(* Logix 5000 AddOnInstructionDefinition export Banner_IOL_QM30VT3_Parameter_v5; software revision 33.00 *)

TYPE Banner_IOL_Device_SubIndex :
STRUCT
   Sub : DINT[34];
END_STRUCT
END_TYPE

TYPE Banner_IOL_Port_v5 :   // UDT that has all of the data items necessary to communicate with a specific Port on a IO-Link Master
STRUCT
   Port_Controlled : INT;   // Each bit represents a port on an IO-Link Master. Set to 1 to tell AOI to control that port.
   Port_Activate : INT;   // Each bit represents a port on an IO-Link Master. When ON that port will process any commands in queue.
   Port_Read : INT;   // Each bit represents a port on an IO-Link Master. Used to determine when device AOI has requested a Read command.
   Port_Write : INT;   // Each bit represents a port on an IO-Link Master. Used to determine when device AOI has requested a Write command.
   Port_RW_Complete : INT;   // Each bit represents a port on an IO-Link Master. Tells device AOI that Read or Write request has been completed.
   Port_Device_Read : INT;
   Data_Transfer : SINT[250];   // Array to transfer data from IO-Master to device AOIs.
END_STRUCT
END_TYPE

TYPE Banner_IOL_QM30VT3_Device :
STRUCT
   Initial_Global_Read : BOOL;
   Command : SINT;
   Data : Banner_IOL_QM30VT3_Device_Index;
   Reset : BOOL;
END_STRUCT
END_TYPE

TYPE Banner_IOL_QM30VT3_Device_Index :
STRUCT
   Index : Banner_IOL_Device_SubIndex[19];
   Metric_Config : Banner_IOL_QM30VT3_Metric_Config;
END_STRUCT
END_TYPE

TYPE Banner_IOL_QM30VT3_Metric_Config :
STRUCT
   Metric_1 : Banner_IOL_QM30VT3_Metric_Data;
   Metric_2 : Banner_IOL_QM30VT3_Metric_Data;
   Metric_3 : Banner_IOL_QM30VT3_Metric_Data;
   Metric_4 : Banner_IOL_QM30VT3_Metric_Data;
   Metric_5 : Banner_IOL_QM30VT3_Metric_Data;
   Metric_6 : Banner_IOL_QM30VT3_Metric_Data;
   Metric_7 : Banner_IOL_QM30VT3_Metric_Data;
   Num_of_Threshold_Samples : DINT;
END_STRUCT
END_TYPE

TYPE Banner_IOL_QM30VT3_Metric_Data :
STRUCT
   Metric : DINT;   // See IODD file for all options.
   Warning_Threshold : REAL;
   Alarm_Treshold : REAL;
END_STRUCT
END_TYPE

TYPE Banner_IOL_Rules :
STRUCT
   Byte_Pos : SINT;   // Byte Position to read from or write data to.
   Multi : SINT;   // Determines if a multiple byte length index is being accessed. Use 2 for 2 bytes length, 3 for 3 byte length, etc..
   Sub_Index : SINT;
   Signed : SINT;   // 0=Unsigned, 1=Signed
END_STRUCT
END_TYPE

TYPE Banner_IOL_Rules_Array :
STRUCT
   Length : DINT;
   Settings : Banner_IOL_Rules_SettingsArray[32];
END_STRUCT
END_TYPE

TYPE Banner_IOL_Rules_SettingsArray :
STRUCT
   Index : DINT;
   Num_Op : INT;   // Number of Operations to read/write Index.
   Total_Bytes : INT;
   RW : SINT;   // 0 = Read Only, 1 = Write Only, 2 = Read or Write
   Rules : Banner_IOL_Rules[34];   // Sub Index Position in IODD.
END_STRUCT
END_TYPE

ADD_ON_INSTRUCTION Banner_IOL_QM30VT3_Parameter_v5   (* revision 5.0 *)
// AOI that reads and writes to an IO-Link devices parameter data.
VAR_IN_OUT
   Device : Banner_IOL_QM30VT3_Device; {required}
   Rules : Banner_IOL_Rules_Array; {required}
   Port_Data : Banner_IOL_Port_v5; {required}
END_VAR
VAR_INPUT
   Port : DINT; {required}
END_VAR
VAR_OUTPUT
   Done : BOOL; {access Read Only, visible}
   Busy : BOOL; {access Read Only, visible}
END_VAR
VAR
   Control : DINT; {access None}
   Inprocess_Index : INT; {access None}
   Index_Write_Inprocess : INT; {access None}
   Index_Write_Control : INT; {access None}
   Global_Read_Command : INT; {access None}
   Command_Being_Processed : BOOL; {access None}
   r_dex2 : INT; {access None}
   r_dex1 : INT; {access None}
   g_index : INT; {access None}
   r_dex3 : INT; {access None}
   r_dex4 : INT; {access None}
   r_dex5 : INT; {access None}
   Wr_Upper : INT; {access None}
   w_dex5 : INT; {access None}
   w_dex4 : INT; {access None}
   w_dex3 : INT; {access None}
   w_dex2 : INT; {access None}
   w_dex1 : INT; {access None}
   m3 : INT; {access None}
   m2 : INT; {access None}
   m1 : INT; {access None}
   s_dex : INT; {access None}
   GlobalCon : DINT; {access None}
   b_dex : INT; {access None}
   Temp_Int : INT; {access None}
END_VAR

ROUTINE Logic   (* ladder *)
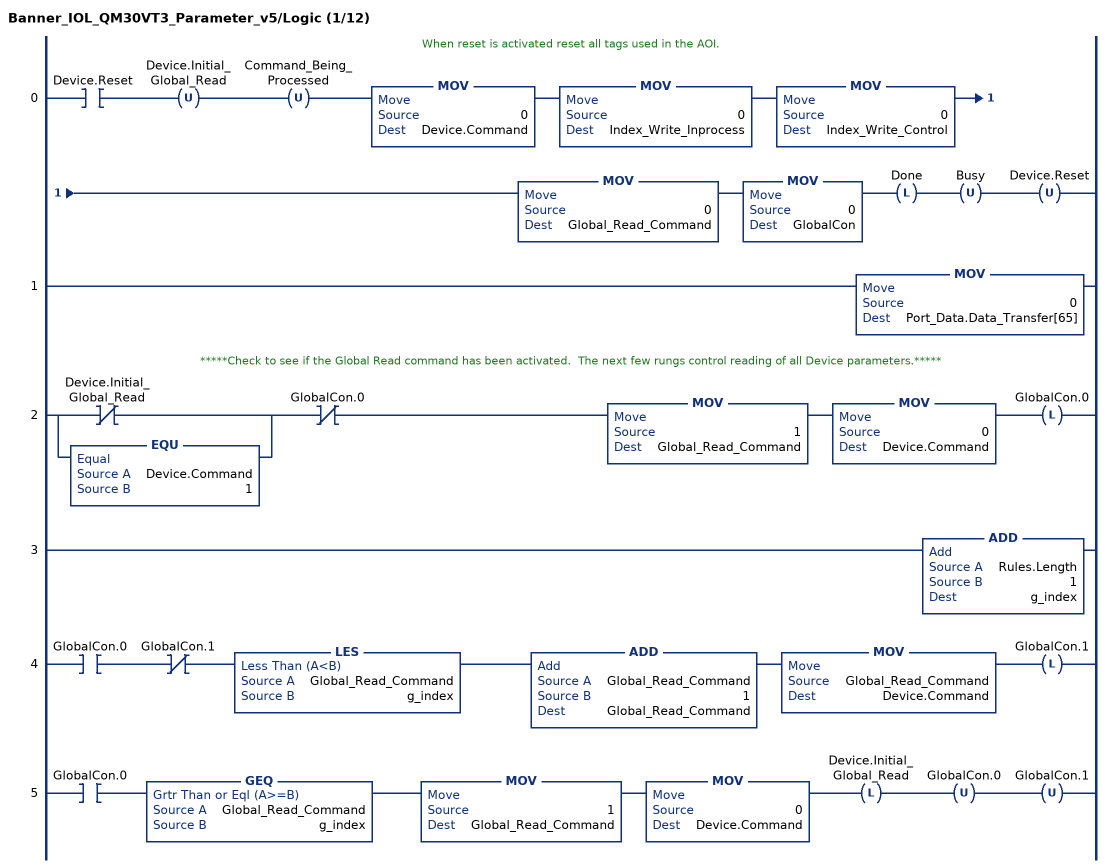
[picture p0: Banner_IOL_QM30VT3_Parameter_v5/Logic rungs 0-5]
   // When reset is activated reset all tags used in the AOI.
   0: XIC(Device.Reset)OTU(Device.Initial_Global_Read)OTU(Command_Being_Processed)MOV(0,Device.Command)MOV(0,Index_Write_Inprocess)MOV(0,Index_Write_Control)MOV(0,Global_Read_Command)MOV(0,GlobalCon)OTL(Done)OTU(Busy)OTU(Device.Reset);
   1: MOV(0,Port_Data.Data_Transfer[65]);
   // *****Check to see if the Global Read command has been activated.  The next few rungs control reading of all Device parameters.*****
   2: [XIO(Device.Initial_Global_Read) ,EQU(Device.Command,1) ]XIO(GlobalCon.0)MOV(1,Global_Read_Command)MOV(0,Device.Command)OTL(GlobalCon.0);
   3: ADD(Rules.Length,1,g_index);
   4: XIC(GlobalCon.0)XIO(GlobalCon.1)LES(Global_Read_Command,g_index)ADD(Global_Read_Command,1,Global_Read_Command)MOV(Global_Read_Command,Device.Command)OTL(GlobalCon.1);
   5: XIC(GlobalCon.0)GEQ(Global_Read_Command,g_index)MOV(1,Global_Read_Command)MOV(0,Device.Command)OTL(Device.Initial_Global_Read)OTU(GlobalCon.0)OTU(GlobalCon.1);
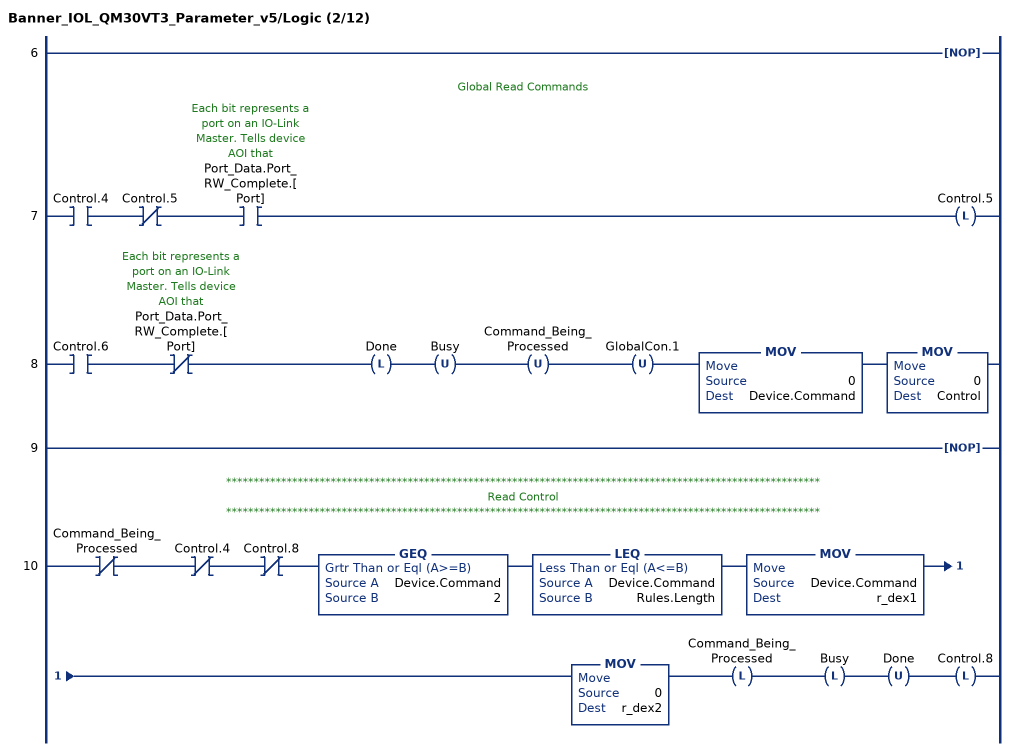
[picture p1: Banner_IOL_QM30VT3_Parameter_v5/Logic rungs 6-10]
   6: NOP();
   // Global Read Commands
   7: XIC(Control.4)XIO(Control.5)XIC(Port_Data.Port_RW_Complete.[Port])OTL(Control.5);
   8: XIC(Control.6)XIO(Port_Data.Port_RW_Complete.[Port])OTL(Done)OTU(Busy)OTU(Command_Being_Processed)OTU(GlobalCon.1)MOV(0,Device.Command)MOV(0,Control);
   9: NOP();
   // ************************************************************************************************************
   // Read Control
   // ************************************************************************************************************
   10: XIO(Command_Being_Processed)XIO(Control.4)XIO(Control.8)GEQ(Device.Command,2)LEQ(Device.Command,Rules.Length)MOV(Device.Command,r_dex1)MOV(0,r_dex2)OTL(Command_Being_Processed)OTL(Busy)OTU(Done)OTL(Control.8);
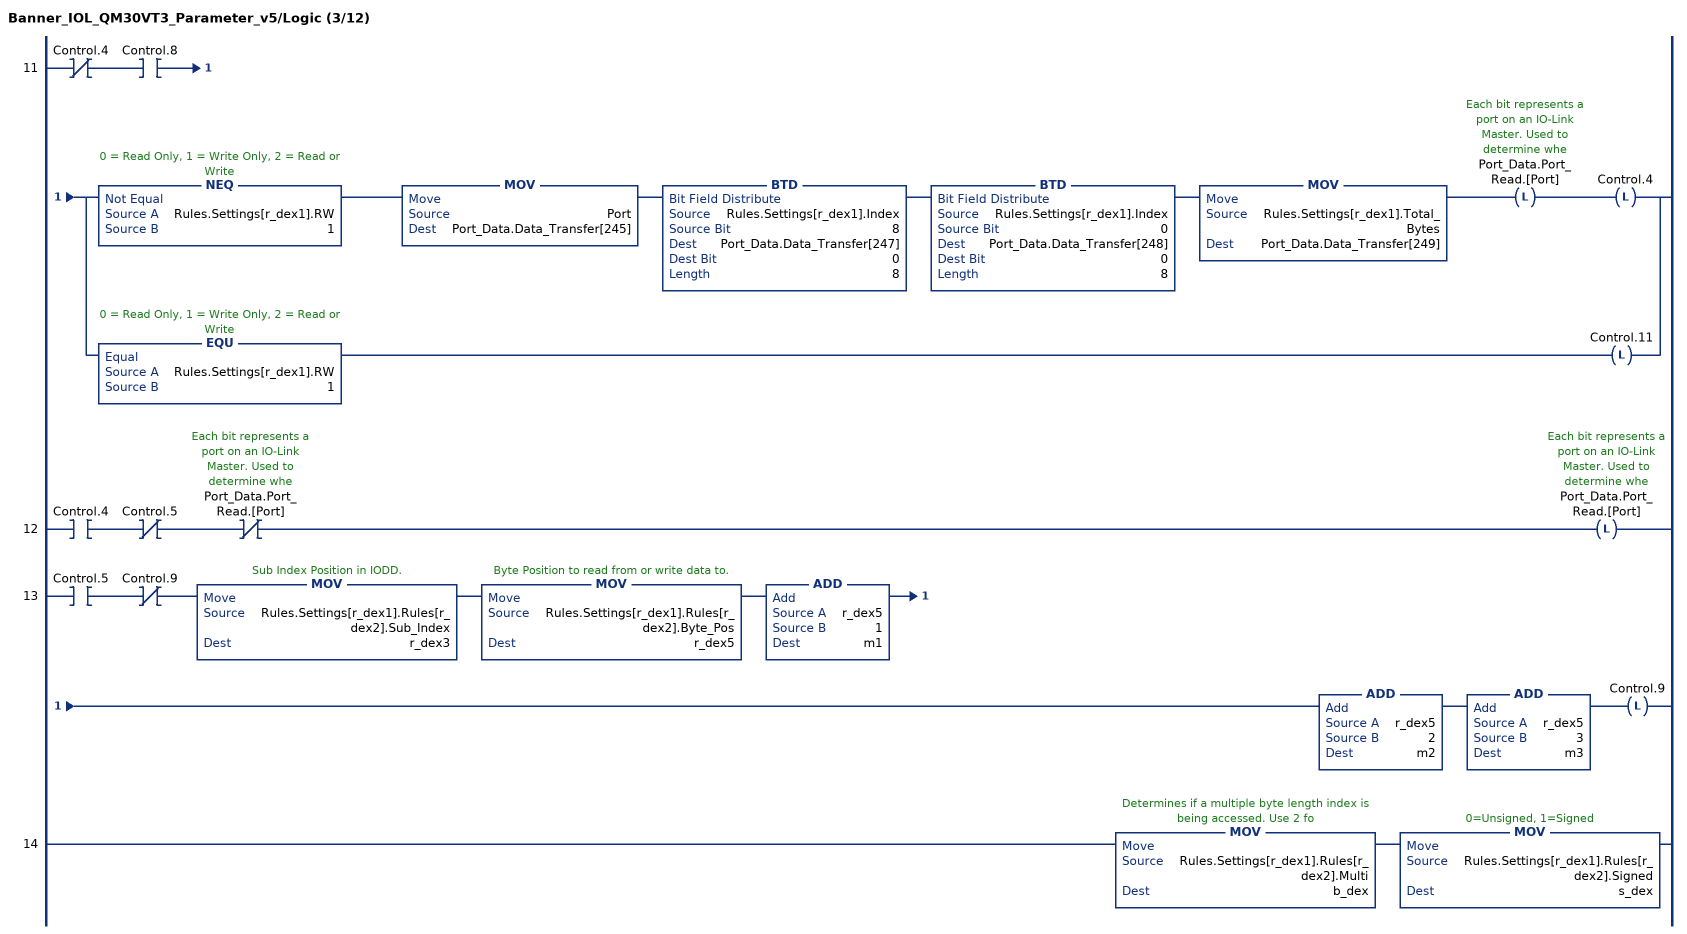
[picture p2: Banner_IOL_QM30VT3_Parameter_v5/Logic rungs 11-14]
   11: XIO(Control.4)XIC(Control.8)[NEQ(Rules.Settings[r_dex1].RW,1) MOV(Port,Port_Data.Data_Transfer[245]) BTD(Rules.Settings[r_dex1].Index,8,Port_Data.Data_Transfer[247],0,8) BTD(Rules.Settings[r_dex1].Index,0,Port_Data.Data_Transfer[248],0,8) MOV(Rules.Settings[r_dex1].Total_Bytes,Port_Data.Data_Transfer[249]) OTL(Port_Data.Port_Read.[Port]) OTL(Control.4) ,EQU(Rules.Settings[r_dex1].RW,1) OTL(Control.11) ];
   12: XIC(Control.4)XIO(Control.5)XIO(Port_Data.Port_Read.[Port])OTL(Port_Data.Port_Read.[Port]);
   13: XIC(Control.5)XIO(Control.9)MOV(Rules.Settings[r_dex1].Rules[r_dex2].Sub_Index,r_dex3)MOV(Rules.Settings[r_dex1].Rules[r_dex2].Byte_Pos,r_dex5)ADD(r_dex5,1,m1)ADD(r_dex5,2,m2)ADD(r_dex5,3,m3)OTL(Control.9);
   14: MOV(Rules.Settings[r_dex1].Rules[r_dex2].Multi,b_dex)MOV(Rules.Settings[r_dex1].Rules[r_dex2].Signed,s_dex);
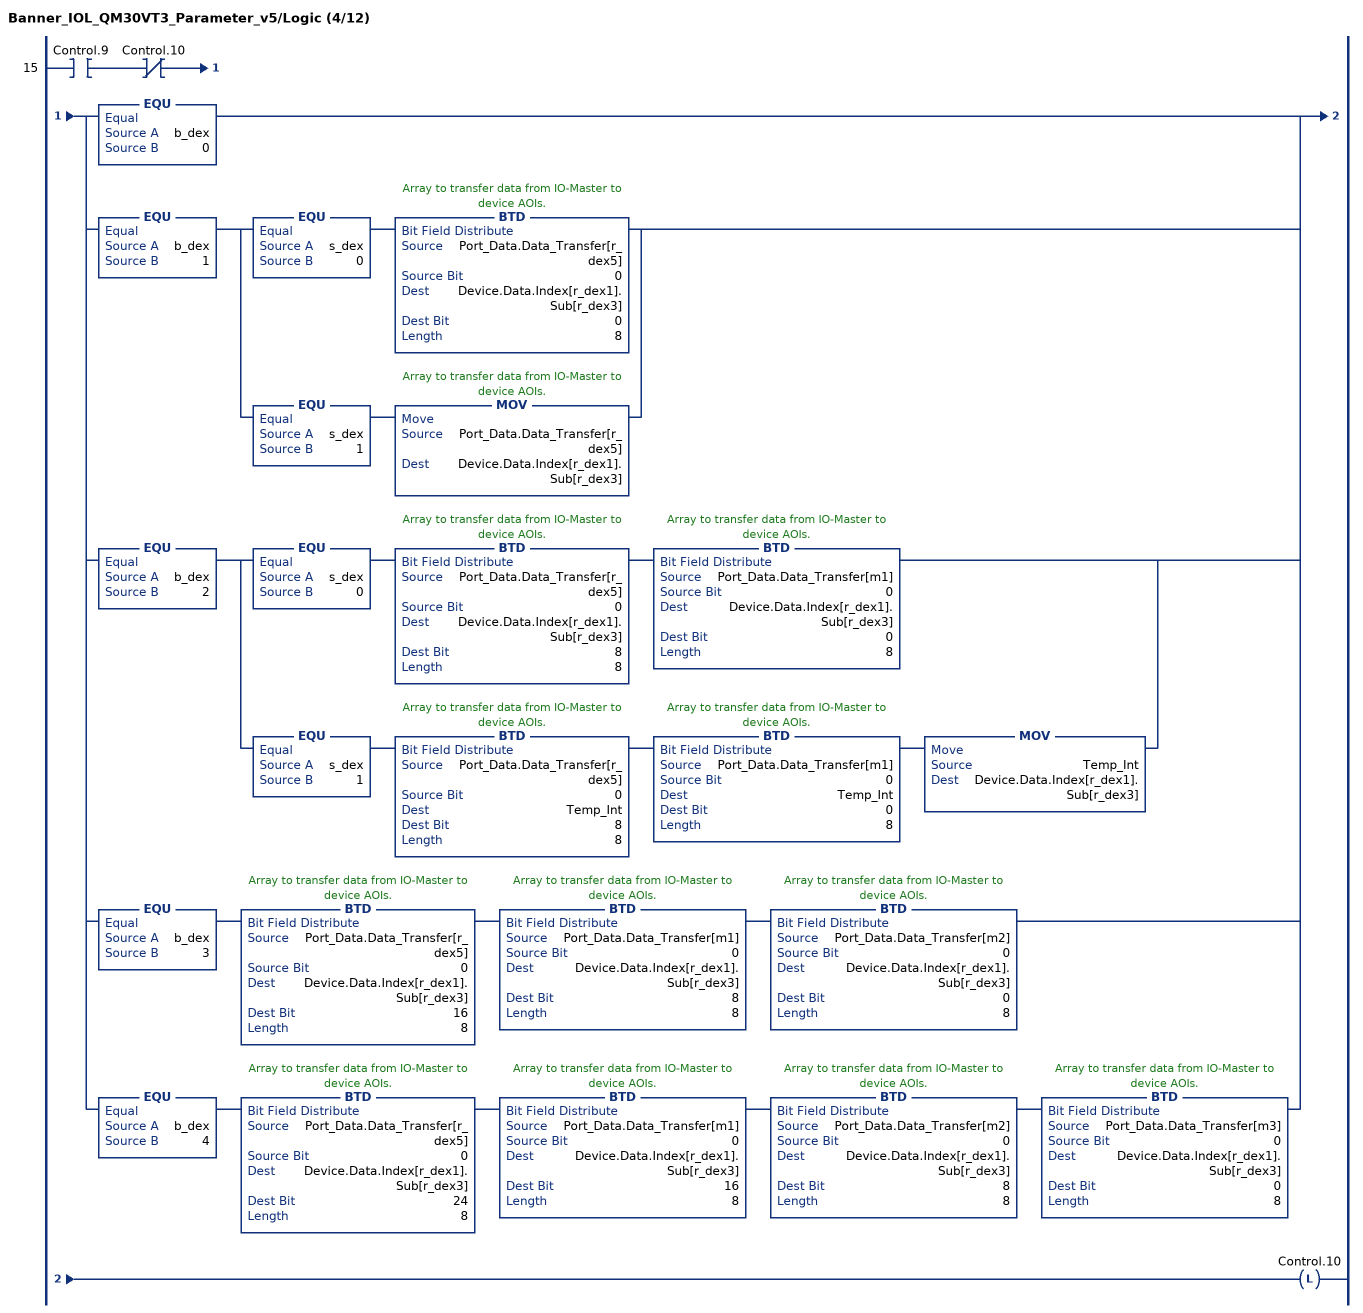
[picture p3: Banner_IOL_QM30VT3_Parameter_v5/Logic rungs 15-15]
   15: XIC(Control.9)XIO(Control.10)[EQU(b_dex,0) ,EQU(b_dex,1) [EQU(s_dex,0) BTD(Port_Data.Data_Transfer[r_dex5],0,Device.Data.Index[r_dex1].Sub[r_dex3],0,8) ,EQU(s_dex,1) MOV(Port_Data.Data_Transfer[r_dex5],Device.Data.Index[r_dex1].Sub[r_dex3]) ] ,EQU(b_dex,2) [EQU(s_dex,0) BTD(Port_Data.Data_Transfer[r_dex5],0,Device.Data.Index[r_dex1].Sub[r_dex3],8,8) BTD(Port_Data.Data_Transfer[m1],0,Device.Data.Index[r_dex1].Sub[r_dex3],0,8) ,EQU(s_dex,1) BTD(Port_Data.Data_Transfer[r_dex5],0,Temp_Int,8,8) BTD(Port_Data.Data_Transfer[m1],0,Temp_Int,0,8) MOV(Temp_Int,Device.Data.Index[r_dex1].Sub[r_dex3]) ] ,EQU(b_dex,3) BTD(Port_Data.Data_Transfer[r_dex5],0,Device.Data.Index[r_dex1].Sub[r_dex3],16,8) BTD(Port_Data.Data_Transfer[m1],0,Device.Data.Index[r_dex1].Sub[r_dex3],8,8) BTD(Port_Data.Data_Transfer[m2],0,Device.Data.Index[r_dex1].Sub[r_dex3],0,8) ,EQU(b_dex,4) BTD(Port_Data.Data_Transfer[r_dex5],0,Device.Data.Index[r_dex1].Sub[r_dex3],24,8) BTD(Port_Data.Data_Transfer[m1],0,Device.Data.Index[r_dex1].Sub[r_dex3],16,8) BTD(Port_Data.Data_Transfer[m2],0,Device.Data.Index[r_dex1].Sub[r_dex3],8,8) BTD(Port_Data.Data_Transfer[m3],0,Device.Data.Index[r_dex1].Sub[r_dex3],0,8) ]OTL(Control.10);
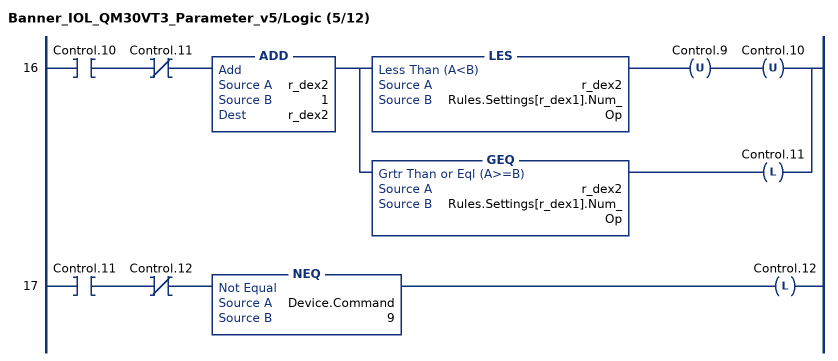
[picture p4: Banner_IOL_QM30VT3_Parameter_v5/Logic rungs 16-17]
   16: XIC(Control.10)XIO(Control.11)ADD(r_dex2,1,r_dex2)[LES(r_dex2,Rules.Settings[r_dex1].Num_Op) OTU(Control.9) OTU(Control.10) ,GEQ(r_dex2,Rules.Settings[r_dex1].Num_Op) OTL(Control.11) ];
   17: XIC(Control.11)XIO(Control.12)NEQ(Device.Command,9)OTL(Control.12);
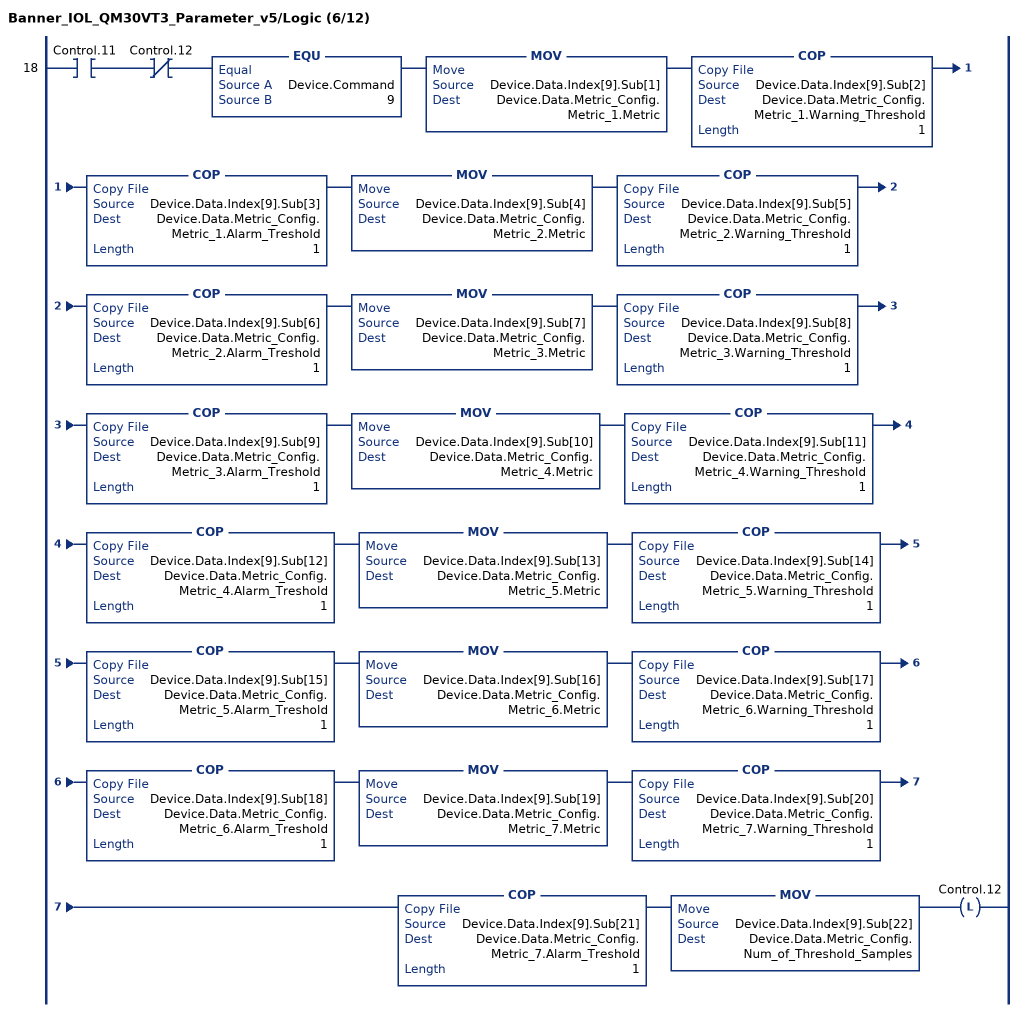
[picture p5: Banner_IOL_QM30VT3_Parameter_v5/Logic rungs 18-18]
   18: XIC(Control.11)XIO(Control.12)EQU(Device.Command,9)MOV(Device.Data.Index[9].Sub[1],Device.Data.Metric_Config.Metric_1.Metric)COP(Device.Data.Index[9].Sub[2],Device.Data.Metric_Config.Metric_1.Warning_Threshold,1)COP(Device.Data.Index[9].Sub[3],Device.Data.Metric_Config.Metric_1.Alarm_Treshold,1)MOV(Device.Data.Index[9].Sub[4],Device.Data.Metric_Config.Metric_2.Metric)COP(Device.Data.Index[9].Sub[5],Device.Data.Metric_Config.Metric_2.Warning_Threshold,1)COP(Device.Data.Index[9].Sub[6],Device.Data.Metric_Config.Metric_2.Alarm_Treshold,1)MOV(Device.Data.Index[9].Sub[7],Device.Data.Metric_Config.Metric_3.Metric)COP(Device.Data.Index[9].Sub[8],Device.Data.Metric_Config.Metric_3.Warning_Threshold,1)COP(Device.Data.Index[9].Sub[9],Device.Data.Metric_Config.Metric_3.Alarm_Treshold,1)MOV(Device.Data.Index[9].Sub[10],Device.Data.Metric_Config.Metric_4.Metric)COP(Device.Data.Index[9].Sub[11],Device.Data.Metric_Config.Metric_4.Warning_Threshold,1)COP(Device.Data.Index[9].Sub[12],Device.Data.Metric_Config.Metric_4.Alarm_Treshold,1)MOV(Device.Data.Index[9].Sub[13],Device.Data.Metric_Config.Metric_5.Metric)COP(Device.Data.Index[9].Sub[14],Device.Data.Metric_Config.Metric_5.Warning_Threshold,1)COP(Device.Data.Index[9].Sub[15],Device.Data.Metric_Config.Metric_5.Alarm_Treshold,1)MOV(Device.Data.Index[9].Sub[16],Device.Data.Metric_Config.Metric_6.Metric)COP(Device.Data.Index[9].Sub[17],Device.Data.Metric_Config.Metric_6.Warning_Threshold,1)COP(Device.Data.Index[9].Sub[18],Device.Data.Metric_Config.Metric_6.Alarm_Treshold,1)MOV(Device.Data.Index[9].Sub[19],Device.Data.Metric_Config.Metric_7.Metric)COP(Device.Data.Index[9].Sub[20],Device.Data.Metric_Config.Metric_7.Warning_Threshold,1)COP(Device.Data.Index[9].Sub[21],Device.Data.Metric_Config.Metric_7.Alarm_Treshold,1)MOV(Device.Data.Index[9].Sub[22],Device.Data.Metric_Config.Num_of_Threshold_Samples)OTL(Control.12);
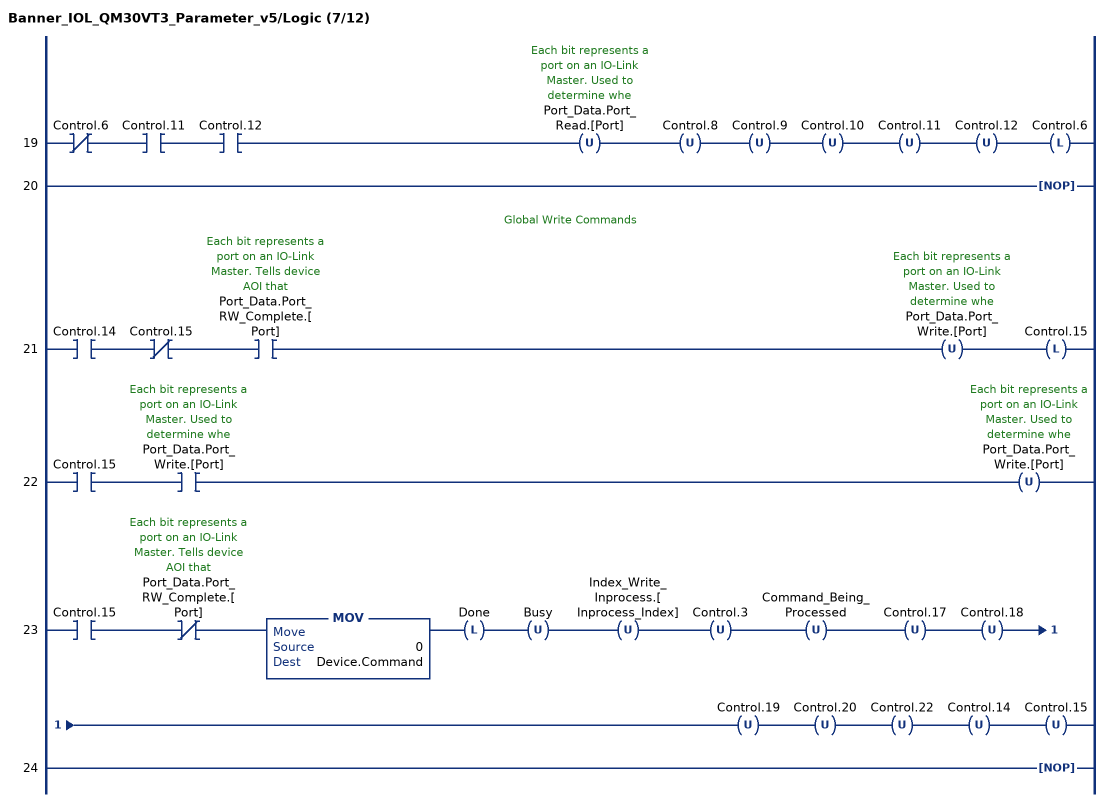
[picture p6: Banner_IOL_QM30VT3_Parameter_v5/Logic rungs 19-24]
   19: XIO(Control.6)XIC(Control.11)XIC(Control.12)OTU(Port_Data.Port_Read.[Port])OTU(Control.8)OTU(Control.9)OTU(Control.10)OTU(Control.11)OTU(Control.12)OTL(Control.6);
   20: NOP();
   // Global Write Commands
   21: XIC(Control.14)XIO(Control.15)XIC(Port_Data.Port_RW_Complete.[Port])OTU(Port_Data.Port_Write.[Port])OTL(Control.15);
   22: XIC(Control.15)XIC(Port_Data.Port_Write.[Port])OTU(Port_Data.Port_Write.[Port]);
   23: XIC(Control.15)XIO(Port_Data.Port_RW_Complete.[Port])MOV(0,Device.Command)OTL(Done)OTU(Busy)OTU(Index_Write_Inprocess.[Inprocess_Index])OTU(Control.3)OTU(Command_Being_Processed)OTU(Control.17)OTU(Control.18)OTU(Control.19)OTU(Control.20)OTU(Control.22)OTU(Control.14)OTU(Control.15);
   24: NOP();
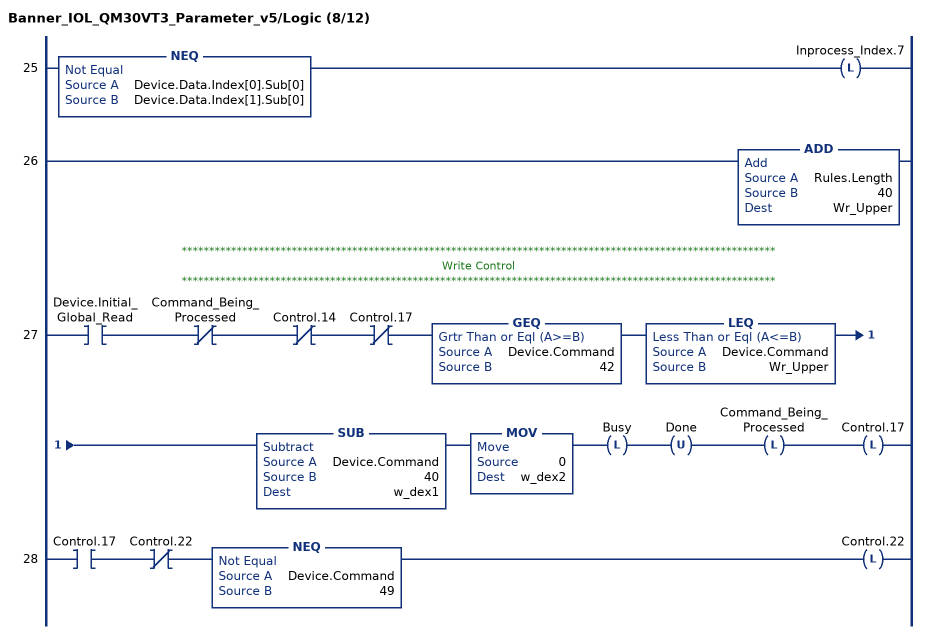
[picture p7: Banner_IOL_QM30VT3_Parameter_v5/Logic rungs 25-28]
   25: NEQ(Device.Data.Index[0].Sub[0],Device.Data.Index[1].Sub[0])OTL(Inprocess_Index.7);
   26: ADD(Rules.Length,40,Wr_Upper);
   // ************************************************************************************************************
   // Write Control
   // ************************************************************************************************************
   27: XIC(Device.Initial_Global_Read)XIO(Command_Being_Processed)XIO(Control.14)XIO(Control.17)GEQ(Device.Command,42)LEQ(Device.Command,Wr_Upper)SUB(Device.Command,40,w_dex1)MOV(0,w_dex2)OTL(Busy)OTU(Done)OTL(Command_Being_Processed)OTL(Control.17);
   28: XIC(Control.17)XIO(Control.22)NEQ(Device.Command,49)OTL(Control.22);
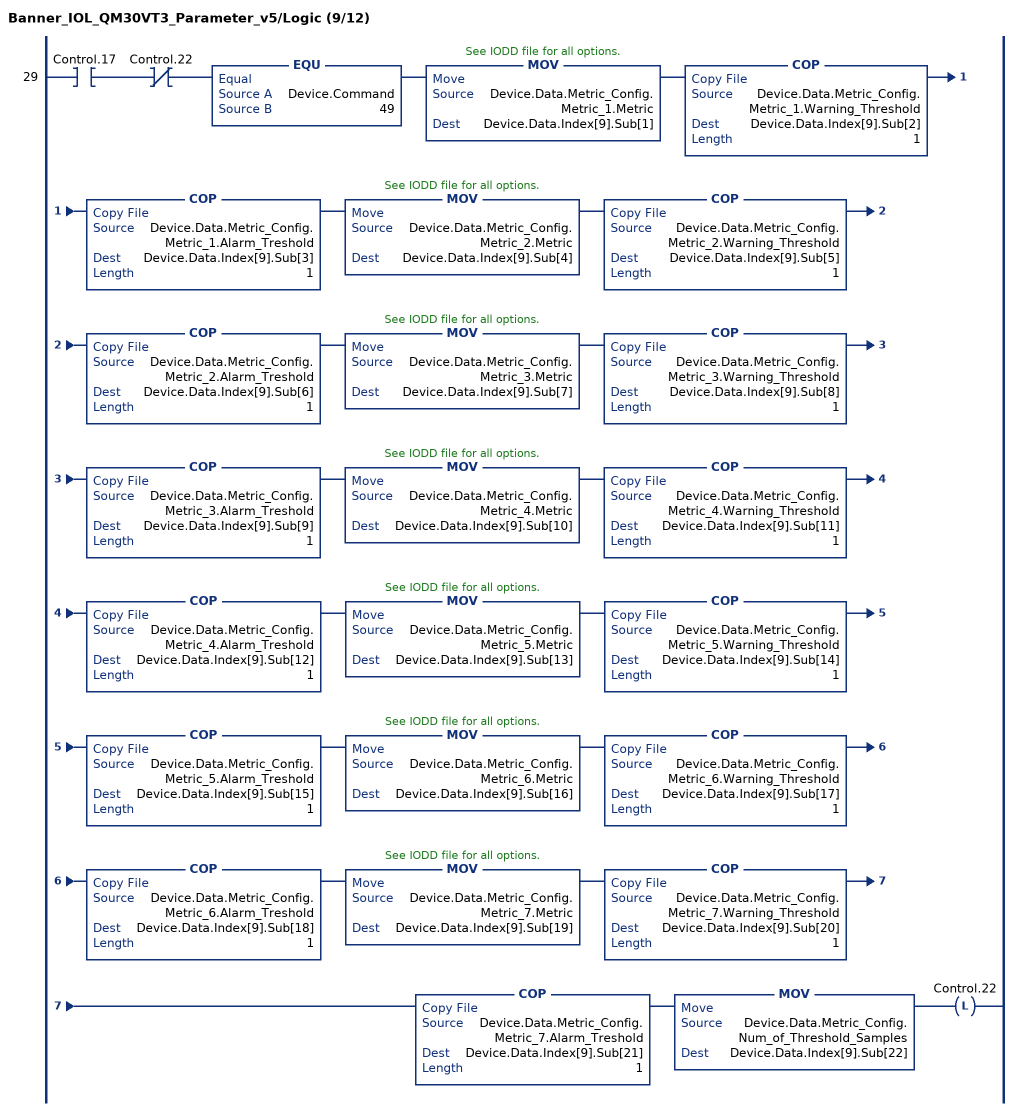
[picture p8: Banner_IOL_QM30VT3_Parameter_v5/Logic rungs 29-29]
   29: XIC(Control.17)XIO(Control.22)EQU(Device.Command,49)MOV(Device.Data.Metric_Config.Metric_1.Metric,Device.Data.Index[9].Sub[1])COP(Device.Data.Metric_Config.Metric_1.Warning_Threshold,Device.Data.Index[9].Sub[2],1)COP(Device.Data.Metric_Config.Metric_1.Alarm_Treshold,Device.Data.Index[9].Sub[3],1)MOV(Device.Data.Metric_Config.Metric_2.Metric,Device.Data.Index[9].Sub[4])COP(Device.Data.Metric_Config.Metric_2.Warning_Threshold,Device.Data.Index[9].Sub[5],1)COP(Device.Data.Metric_Config.Metric_2.Alarm_Treshold,Device.Data.Index[9].Sub[6],1)MOV(Device.Data.Metric_Config.Metric_3.Metric,Device.Data.Index[9].Sub[7])COP(Device.Data.Metric_Config.Metric_3.Warning_Threshold,Device.Data.Index[9].Sub[8],1)COP(Device.Data.Metric_Config.Metric_3.Alarm_Treshold,Device.Data.Index[9].Sub[9],1)MOV(Device.Data.Metric_Config.Metric_4.Metric,Device.Data.Index[9].Sub[10])COP(Device.Data.Metric_Config.Metric_4.Warning_Threshold,Device.Data.Index[9].Sub[11],1)COP(Device.Data.Metric_Config.Metric_4.Alarm_Treshold,Device.Data.Index[9].Sub[12],1)MOV(Device.Data.Metric_Config.Metric_5.Metric,Device.Data.Index[9].Sub[13])COP(Device.Data.Metric_Config.Metric_5.Warning_Threshold,Device.Data.Index[9].Sub[14],1)COP(Device.Data.Metric_Config.Metric_5.Alarm_Treshold,Device.Data.Index[9].Sub[15],1)MOV(Device.Data.Metric_Config.Metric_6.Metric,Device.Data.Index[9].Sub[16])COP(Device.Data.Metric_Config.Metric_6.Warning_Threshold,Device.Data.Index[9].Sub[17],1)COP(Device.Data.Metric_Config.Metric_6.Alarm_Treshold,Device.Data.Index[9].Sub[18],1)MOV(Device.Data.Metric_Config.Metric_7.Metric,Device.Data.Index[9].Sub[19])COP(Device.Data.Metric_Config.Metric_7.Warning_Threshold,Device.Data.Index[9].Sub[20],1)COP(Device.Data.Metric_Config.Metric_7.Alarm_Treshold,Device.Data.Index[9].Sub[21],1)MOV(Device.Data.Metric_Config.Num_of_Threshold_Samples,Device.Data.Index[9].Sub[22])OTL(Control.22);
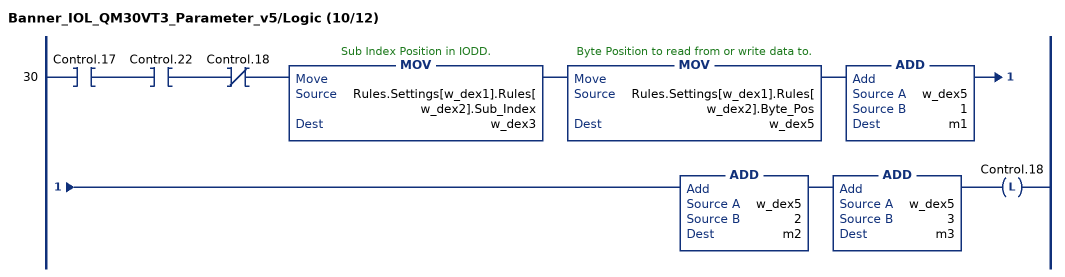
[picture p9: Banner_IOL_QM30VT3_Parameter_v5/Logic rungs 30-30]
   30: XIC(Control.17)XIC(Control.22)XIO(Control.18)MOV(Rules.Settings[w_dex1].Rules[w_dex2].Sub_Index,w_dex3)MOV(Rules.Settings[w_dex1].Rules[w_dex2].Byte_Pos,w_dex5)ADD(w_dex5,1,m1)ADD(w_dex5,2,m2)ADD(w_dex5,3,m3)OTL(Control.18);
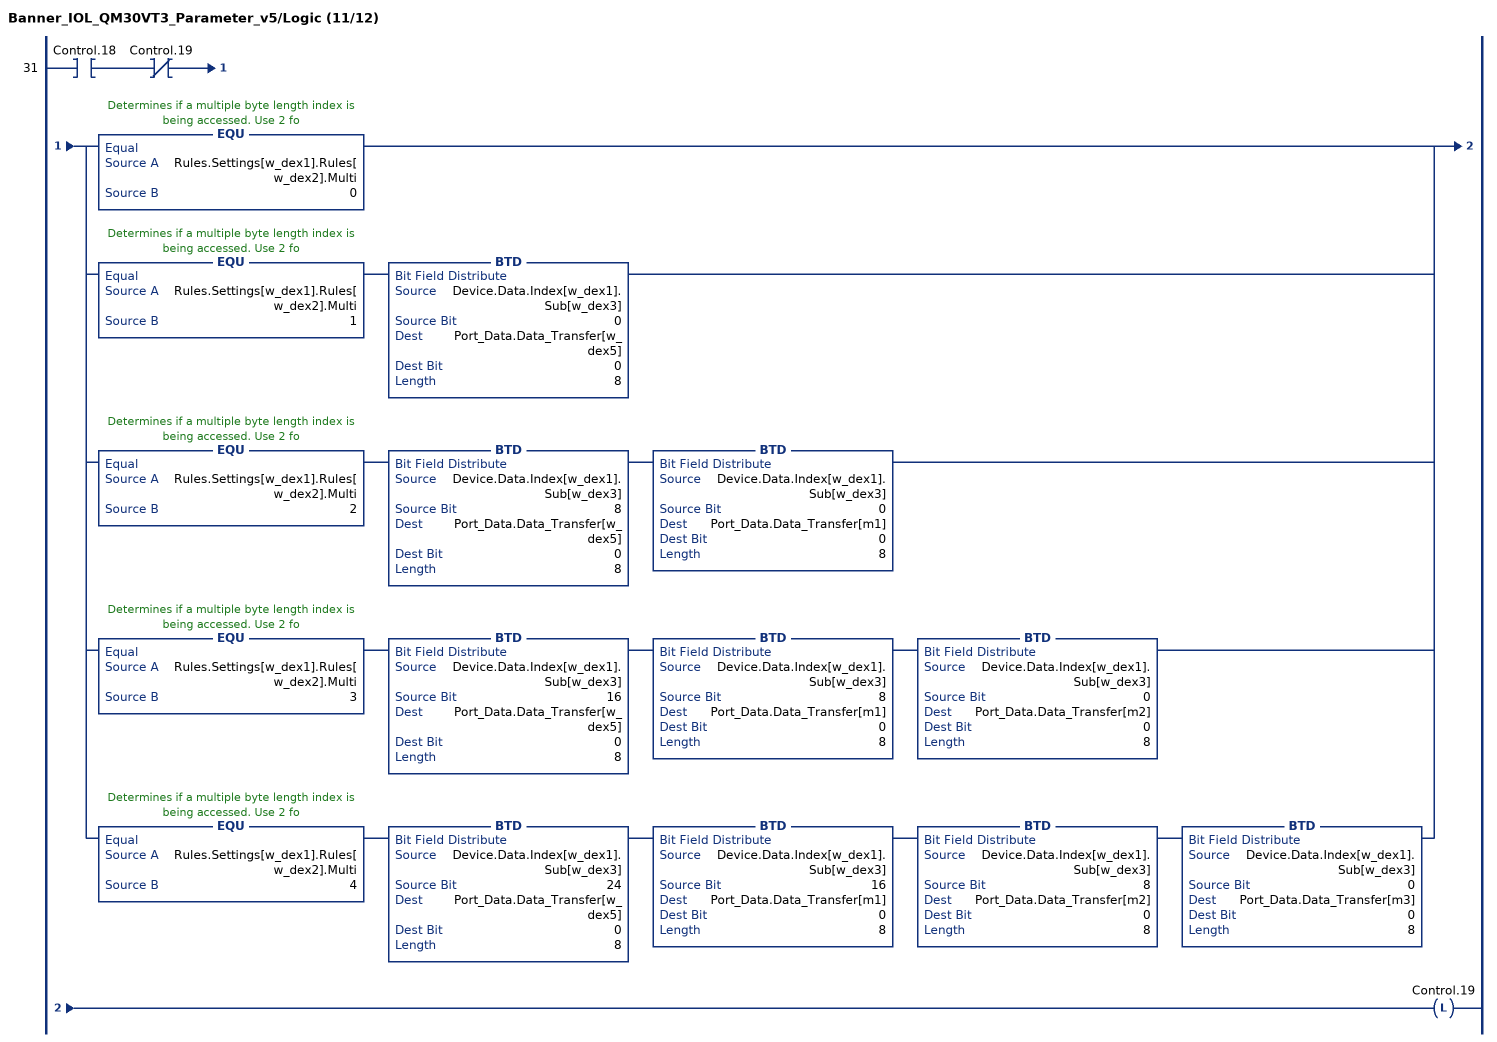
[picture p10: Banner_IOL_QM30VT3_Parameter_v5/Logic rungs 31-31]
   31: XIC(Control.18)XIO(Control.19)[EQU(Rules.Settings[w_dex1].Rules[w_dex2].Multi,0) ,EQU(Rules.Settings[w_dex1].Rules[w_dex2].Multi,1) BTD(Device.Data.Index[w_dex1].Sub[w_dex3],0,Port_Data.Data_Transfer[w_dex5],0,8) ,EQU(Rules.Settings[w_dex1].Rules[w_dex2].Multi,2) BTD(Device.Data.Index[w_dex1].Sub[w_dex3],8,Port_Data.Data_Transfer[w_dex5],0,8) BTD(Device.Data.Index[w_dex1].Sub[w_dex3],0,Port_Data.Data_Transfer[m1],0,8) ,EQU(Rules.Settings[w_dex1].Rules[w_dex2].Multi,3) BTD(Device.Data.Index[w_dex1].Sub[w_dex3],16,Port_Data.Data_Transfer[w_dex5],0,8) BTD(Device.Data.Index[w_dex1].Sub[w_dex3],8,Port_Data.Data_Transfer[m1],0,8) BTD(Device.Data.Index[w_dex1].Sub[w_dex3],0,Port_Data.Data_Transfer[m2],0,8) ,EQU(Rules.Settings[w_dex1].Rules[w_dex2].Multi,4) BTD(Device.Data.Index[w_dex1].Sub[w_dex3],24,Port_Data.Data_Transfer[w_dex5],0,8) BTD(Device.Data.Index[w_dex1].Sub[w_dex3],16,Port_Data.Data_Transfer[m1],0,8) BTD(Device.Data.Index[w_dex1].Sub[w_dex3],8,Port_Data.Data_Transfer[m2],0,8) BTD(Device.Data.Index[w_dex1].Sub[w_dex3],0,Port_Data.Data_Transfer[m3],0,8) ]OTL(Control.19);
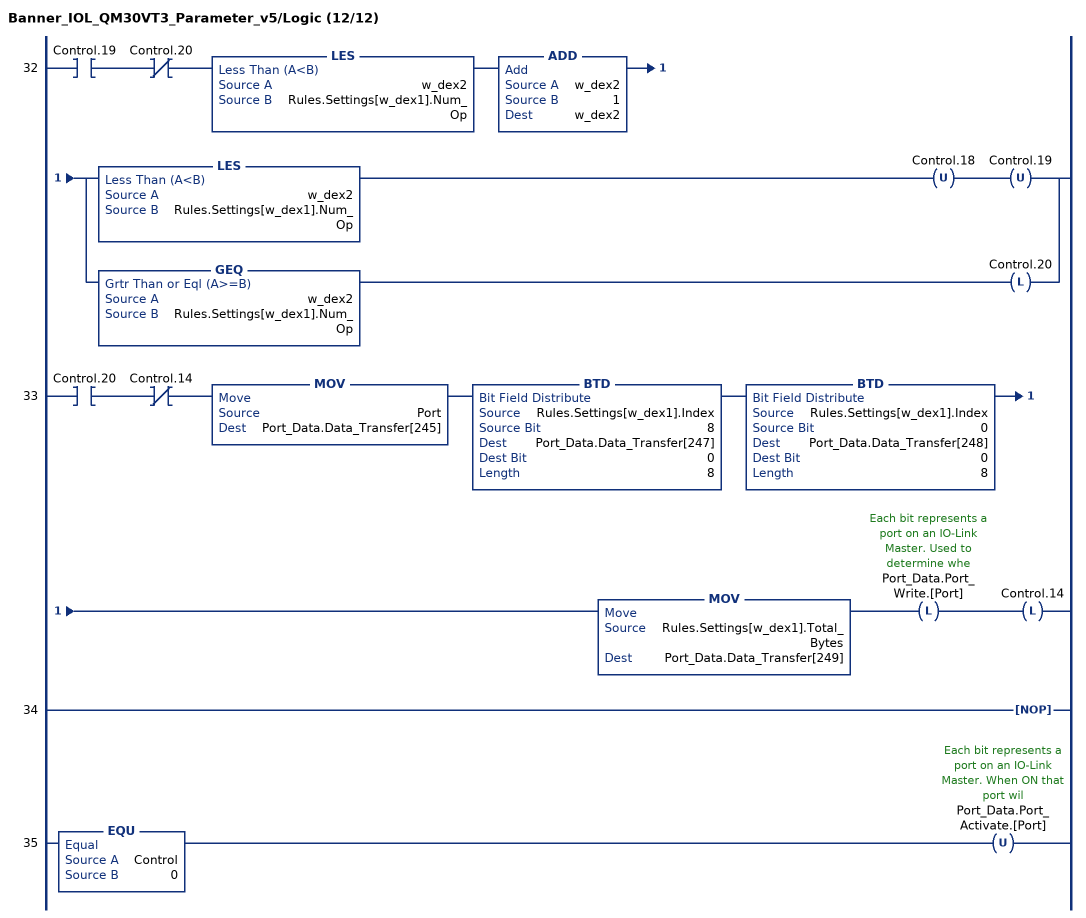
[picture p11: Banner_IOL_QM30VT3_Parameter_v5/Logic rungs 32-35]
   32: XIC(Control.19)XIO(Control.20)LES(w_dex2,Rules.Settings[w_dex1].Num_Op)ADD(w_dex2,1,w_dex2)[LES(w_dex2,Rules.Settings[w_dex1].Num_Op) OTU(Control.18) OTU(Control.19) ,GEQ(w_dex2,Rules.Settings[w_dex1].Num_Op) OTL(Control.20) ];
   33: XIC(Control.20)XIO(Control.14)MOV(Port,Port_Data.Data_Transfer[245])BTD(Rules.Settings[w_dex1].Index,8,Port_Data.Data_Transfer[247],0,8)BTD(Rules.Settings[w_dex1].Index,0,Port_Data.Data_Transfer[248],0,8)MOV(Rules.Settings[w_dex1].Total_Bytes,Port_Data.Data_Transfer[249])OTL(Port_Data.Port_Write.[Port])OTL(Control.14);
   34: NOP();
   35: EQU(Control,0)OTU(Port_Data.Port_Activate.[Port]);
END_ROUTINE
END_ADD_ON_INSTRUCTION
